(* Logix 5000 AddOnInstructionDefinition export SPEL_LocalSet; software revision 30.01 *)

ADD_ON_INSTRUCTION SPEL_ExecCmd   (* revision 1.2 *)
// Executes a command in the robot controller.  Normally this is called by higher level AOIs.
VAR_INPUT
   Start : BOOL; {required}
   MaxTime : DINT := 3000; {required}
END_VAR
VAR_OUTPUT
   InCycle : BOOL; {access Read Only, visible}
   Done : BOOL; {access Read Only, visible}
   Error : BOOL; {access Read Only, visible}
END_VAR
VAR_IN_OUT
   ExtInputs : AB:ETHERNET_MODULE_INT_128Bytes:I:0; {required}
        .DATA[0].0   // ExtCmdGet
        .DATA[0].1   // ExtRespSet
        .DATA[0].2   // ExtCmdResult
        .DATA[0].3   // ExtError
   ExtOutputs : AB:ETHERNET_MODULE_INT_128Bytes:O:0; {required}
        .DATA[0].0   // ExtCmdSet
        .DATA[0].1   // ExtRespGet
        .DATA[0].2   // ExtCmdReset
END_VAR
VAR_INPUT
   Cmd : INT; {required}
   CmdParam1 : INT; {required}
   CmdParam2 : INT; {required}
   CmdParam3 : INT; {required}
   CmdParam4 : INT; {required}
   CmdParam5 : INT; {required}
   CmdParam6 : INT; {required}
   CmdParam7 : INT; {required}
END_VAR
VAR_OUTPUT
   CmdEcho : INT; {access Read Only, visible}
   Resp1 : INT; {access Read Only, visible}
   Resp2 : INT; {access Read Only, visible}
   Resp3 : INT; {access Read Only, visible}
   Resp4 : INT; {access Read Only, visible}
   Resp5 : INT; {access Read Only, visible}
   Resp6 : INT; {access Read Only, visible}
   Resp7 : INT; {access Read Only, visible}
   ErrCode1 : INT; {access Read Only, visible}
   ErrCode2 : INT; {access Read Only, visible}
END_VAR
VAR
   ExtReset : BOOL; {access None}
   ExtError : BOOL; {access None}
   ExtCmdSet : BOOL; {access None}   // Cmd Ready
   ExtCmdGet : BOOL; {access None}   // Cmd Received
   CmdXferDone : BOOL; {access None}
   ExtRespSet : BOOL; {access None}   // Resp Ready
   RespXferDone : BOOL; {access None}
   ExtCmdResult : BOOL; {access None}   // Normal or Error?
   TmrCmdDataRdy : TIMER := (PRE := 5); {access None}
   OneShotDoneOff : BOOL; {access None}
   OneShotStart : BOOL; {access None}
   StartInit : BOOL; {access None}
   OneShotStartError : BOOL; {access None}
   TmrCycle : TIMER := (PRE := 5000); {access None}
   OneshotTmrPreset : BOOL; {access None}
   TmrCmdSet : TIMER := (PRE := 20); {access None}
   OnShotCmdDataXfer : BOOL; {access None}
   OneShotRespDataXfer : BOOL; {access None}
   OneShotDataRdy : BOOL; {access None}
   OtherCmdInCycle : BOOL; {access None}
   s : BOOL; {access None}
   OneShotUnsetCmdIncycle : BOOL; {access None}
   OneShotSetCmdIncycle : BOOL; {access None}
   OneShotSetOtherCmdInCycleError : BOOL; {access None}
   OneShotSetBit : BOOL; {access None}
   MaxTimeError : BOOL; {access None}
END_VAR

ROUTINE Logic   (* ladder *)
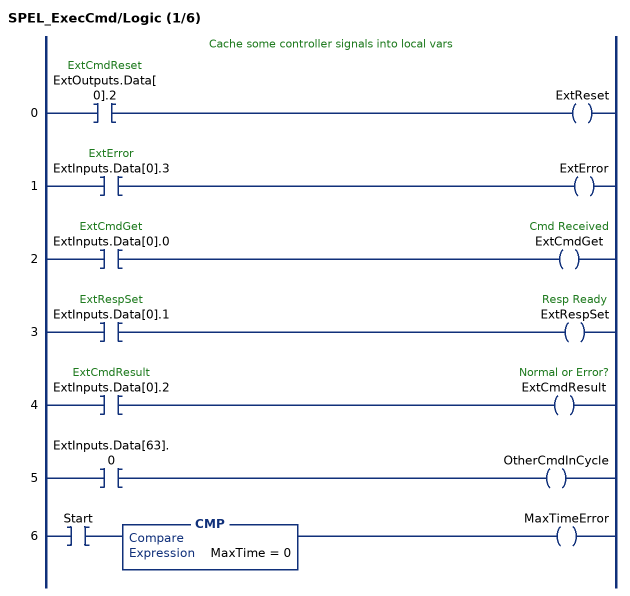
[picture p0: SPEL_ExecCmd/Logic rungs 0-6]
   // Cache some controller signals into local vars
   0: XIC(ExtOutputs.Data[0].2)OTE(ExtReset);
   1: XIC(ExtInputs.Data[0].3)OTE(ExtError);
   2: XIC(ExtInputs.Data[0].0)OTE(ExtCmdGet);
   3: XIC(ExtInputs.Data[0].1)OTE(ExtRespSet);
   4: XIC(ExtInputs.Data[0].2)OTE(ExtCmdResult);
   5: XIC(ExtInputs.Data[63].0)OTE(OtherCmdInCycle);
   6: XIC(Start)CMP(MaxTime = 0)OTE(MaxTimeError);
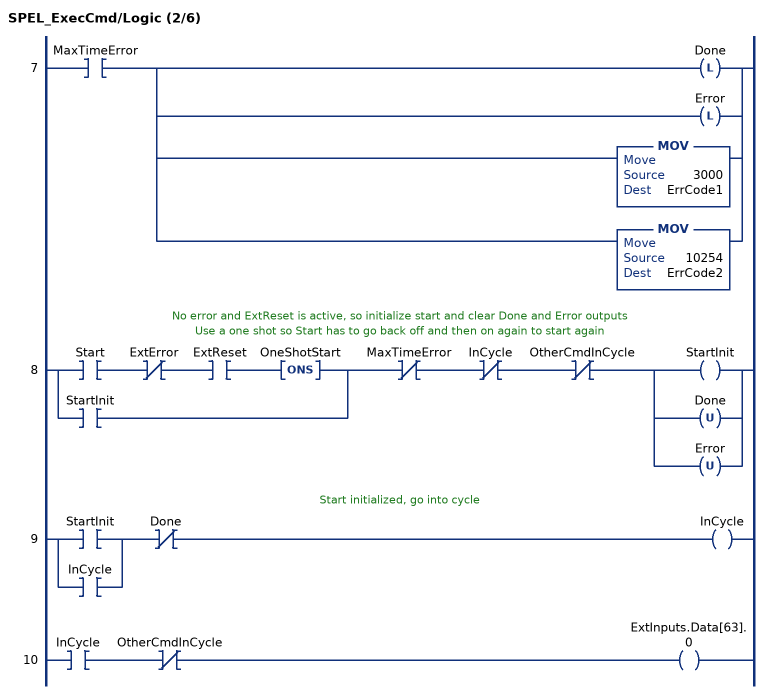
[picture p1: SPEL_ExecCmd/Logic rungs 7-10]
   7: XIC(MaxTimeError)[OTL(Done) ,OTL(Error) ,MOV(3000,ErrCode1) ,MOV(10254,ErrCode2) ];
   // No error and ExtReset is active, so initialize start and clear Done and Error outputs
   // Use a one shot so Start has to go back off and then on again to start again
   8: [XIC(Start) XIO(ExtError) XIC(ExtReset) ONS(OneShotStart) ,XIC(StartInit) ]XIO(MaxTimeError)XIO(InCycle)XIO(OtherCmdInCycle)[OTE(StartInit) ,OTU(Done) ,OTU(Error) ];
   // Start initialized, go into cycle
   9: [XIC(StartInit) ,XIC(InCycle) ]XIO(Done)OTE(InCycle);
   10: XIC(InCycle)XIO(OtherCmdInCycle)OTE(ExtInputs.Data[63].0);
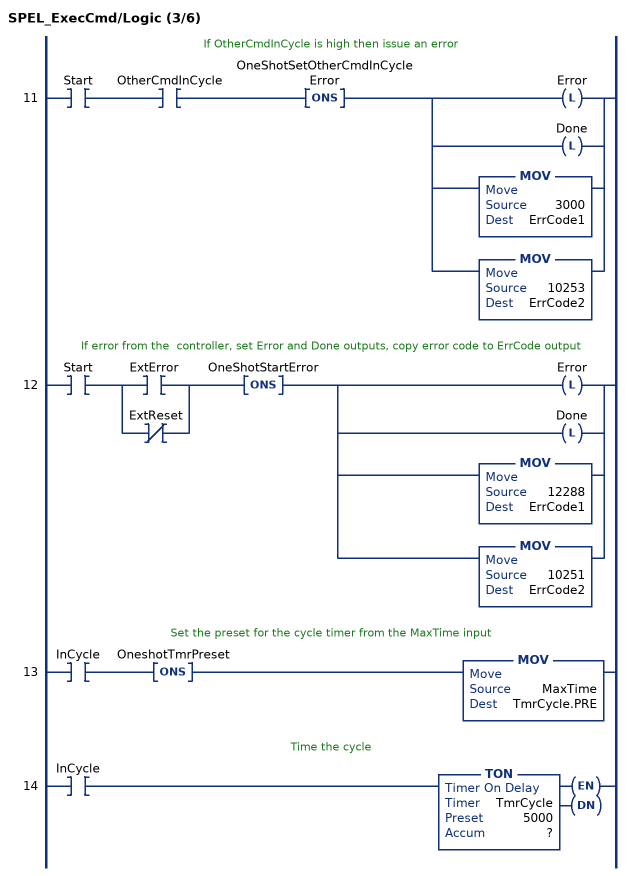
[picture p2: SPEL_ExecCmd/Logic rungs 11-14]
   // If OtherCmdInCycle is high then issue an error
   11: XIC(Start)XIC(OtherCmdInCycle)ONS(OneShotSetOtherCmdInCycleError)[OTL(Error) ,OTL(Done) ,MOV(3000,ErrCode1) ,MOV(10253,ErrCode2) ];
   // If error from the  controller, set Error and Done outputs, copy error code to ErrCode output
   12: XIC(Start)[XIC(ExtError) ,XIO(ExtReset) ]ONS(OneShotStartError)[OTL(Error) ,OTL(Done) ,MOV(12288,ErrCode1) ,MOV(10251,ErrCode2) ];
   // Set the preset for the cycle timer from the MaxTime input
   13: XIC(InCycle)ONS(OneshotTmrPreset)MOV(MaxTime,TmrCycle.PRE);
   // Time the cycle
   14: XIC(InCycle)TON(TmrCycle,?,?);
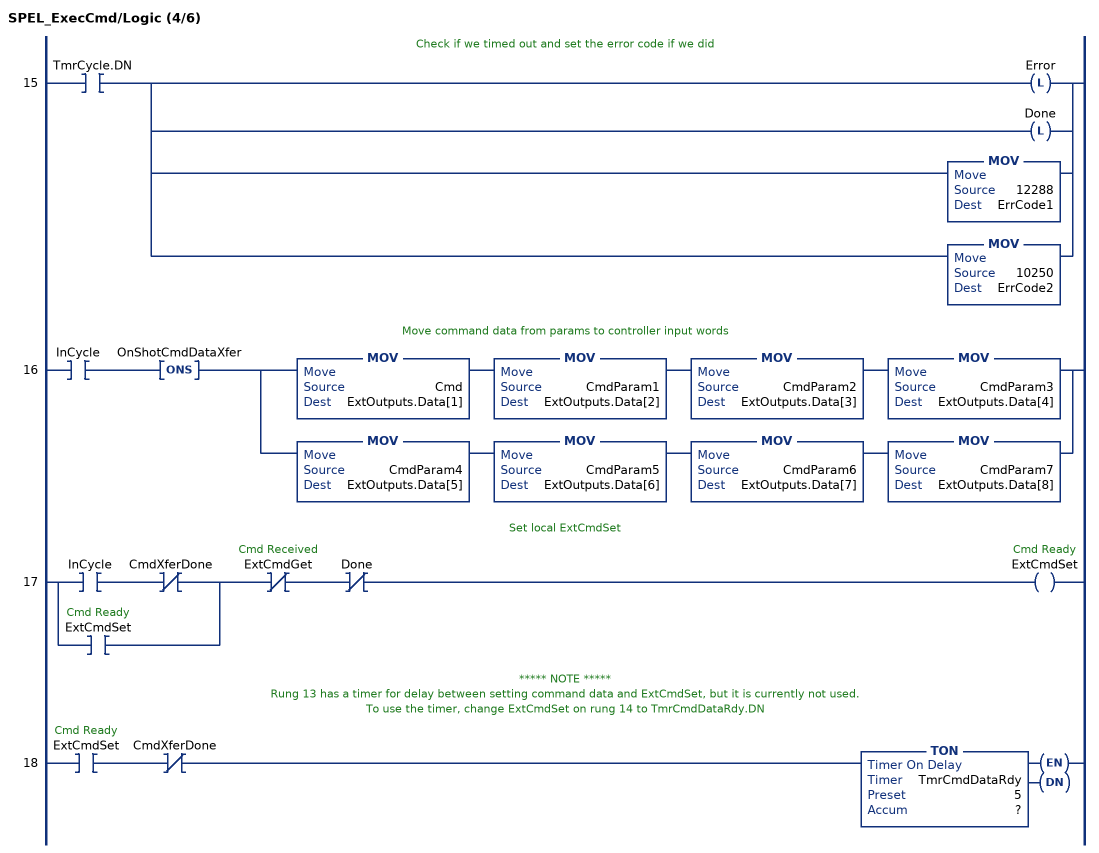
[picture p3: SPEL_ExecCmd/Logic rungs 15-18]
   // Check if we timed out and set the error code if we did
   15: XIC(TmrCycle.DN)[OTL(Error) ,OTL(Done) ,MOV(12288,ErrCode1) ,MOV(10250,ErrCode2) ];
   // Move command data from params to controller input words
   16: XIC(InCycle)ONS(OnShotCmdDataXfer)[MOV(Cmd,ExtOutputs.Data[1]) MOV(CmdParam1,ExtOutputs.Data[2]) MOV(CmdParam2,ExtOutputs.Data[3]) MOV(CmdParam3,ExtOutputs.Data[4]) ,MOV(CmdParam4,ExtOutputs.Data[5]) MOV(CmdParam5,ExtOutputs.Data[6]) MOV(CmdParam6,ExtOutputs.Data[7]) MOV(CmdParam7,ExtOutputs.Data[8]) ];
   // Set local ExtCmdSet
   17: [XIC(InCycle) XIO(CmdXferDone) ,XIC(ExtCmdSet) ]XIO(ExtCmdGet)XIO(Done)OTE(ExtCmdSet);
   // ***** NOTE *****
   // Rung 13 has a timer for delay between setting command data and ExtCmdSet, but it is currently not used.
   // To use the timer, change ExtCmdSet on rung 14 to TmrCmdDataRdy.DN
   18: XIC(ExtCmdSet)XIO(CmdXferDone)TON(TmrCmdDataRdy,?,?);
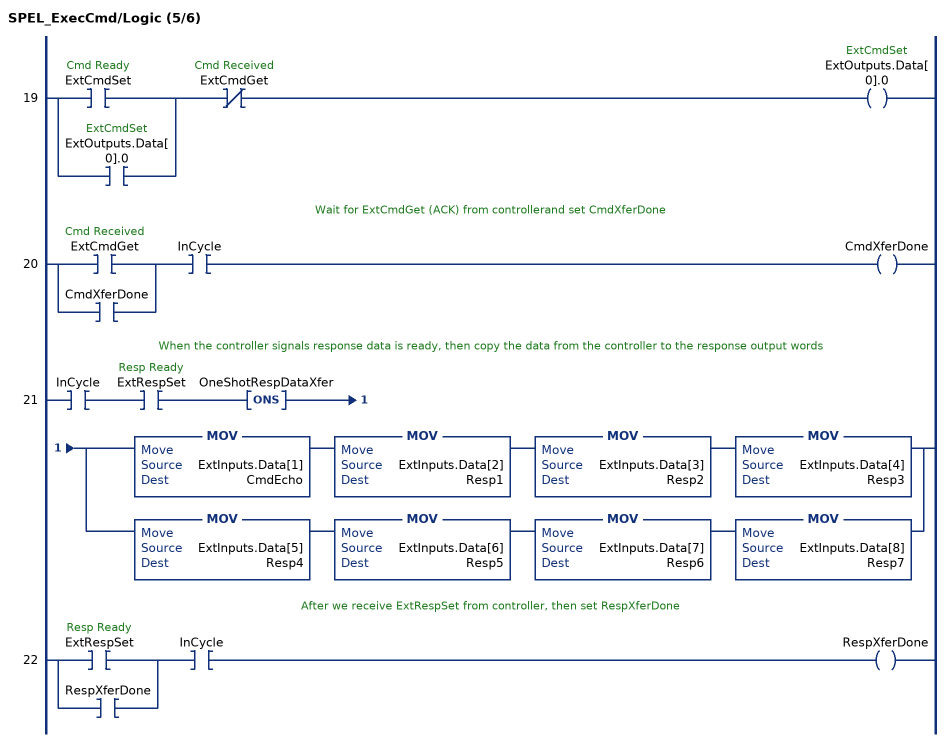
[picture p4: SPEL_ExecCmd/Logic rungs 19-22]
   19: [XIC(ExtCmdSet) ,XIC(ExtOutputs.Data[0].0) ]XIO(ExtCmdGet)OTE(ExtOutputs.Data[0].0);
   // Wait for ExtCmdGet (ACK) from controllerand set CmdXferDone
   20: [XIC(ExtCmdGet) ,XIC(CmdXferDone) ]XIC(InCycle)OTE(CmdXferDone);
   // When the controller signals response data is ready, then copy the data from the controller to the response output words
   21: XIC(InCycle)XIC(ExtRespSet)ONS(OneShotRespDataXfer)[MOV(ExtInputs.Data[1],CmdEcho) MOV(ExtInputs.Data[2],Resp1) MOV(ExtInputs.Data[3],Resp2) MOV(ExtInputs.Data[4],Resp3) ,MOV(ExtInputs.Data[5],Resp4) MOV(ExtInputs.Data[6],Resp5) MOV(ExtInputs.Data[7],Resp6) MOV(ExtInputs.Data[8],Resp7) ];
   // After we receive ExtRespSet from controller, then set RespXferDone
   22: [XIC(ExtRespSet) ,XIC(RespXferDone) ]XIC(InCycle)OTE(RespXferDone);
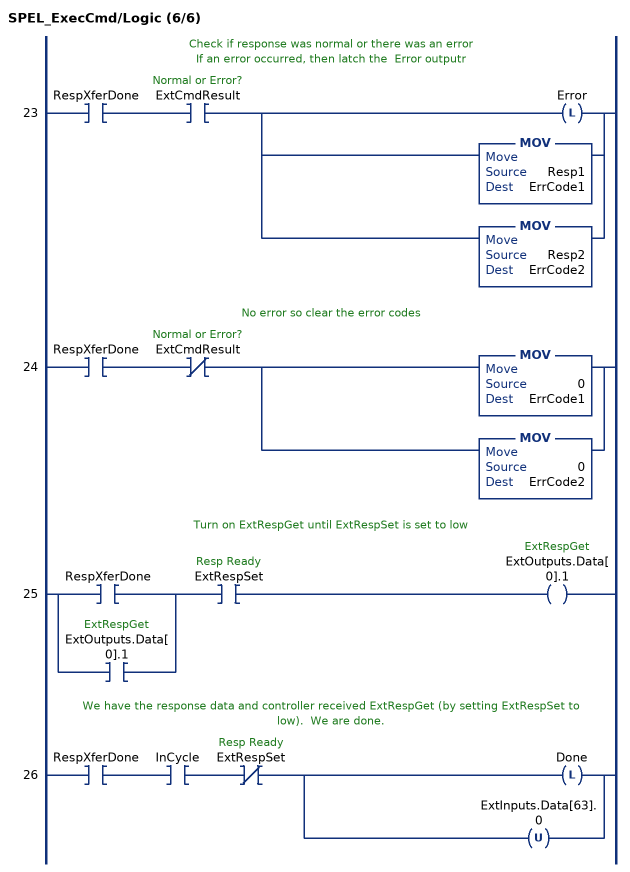
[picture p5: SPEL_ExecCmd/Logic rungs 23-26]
   // Check if response was normal or there was an error
   // If an error occurred, then latch the  Error outputr
   23: XIC(RespXferDone)XIC(ExtCmdResult)[OTL(Error) ,MOV(Resp1,ErrCode1) ,MOV(Resp2,ErrCode2) ];
   // No error so clear the error codes
   24: XIC(RespXferDone)XIO(ExtCmdResult)[MOV(0,ErrCode1) ,MOV(0,ErrCode2) ];
   // Turn on ExtRespGet until ExtRespSet is set to low
   25: [XIC(RespXferDone) ,XIC(ExtOutputs.Data[0].1) ]XIC(ExtRespSet)OTE(ExtOutputs.Data[0].1);
   // We have the response data and controller received ExtRespGet (by setting ExtRespSet to low).  We are done.
   26: XIC(RespXferDone)XIC(InCycle)XIO(ExtRespSet)[OTL(Done) ,OTU(ExtInputs.Data[63].0) ];
END_ROUTINE
END_ADD_ON_INSTRUCTION

ADD_ON_INSTRUCTION SPEL_LocalSet   (* revision 1.2, vendor SEIKO EPSON CORP. *)
// Sets the local coordinate system of the specified coordinate number by each coordinate.
VAR_INPUT
   Start : BOOL; {required}
END_VAR
VAR_OUTPUT
   InCycle : BOOL; {access Read Only, visible}
   Done : BOOL; {access Read Only, visible}
   Error : BOOL; {access Read Only, visible}
END_VAR
VAR_INPUT
   NumAxes : INT; {required}
   LocalNum : INT; {required}
   LocalX : REAL; {required}
   LocalY : REAL; {required}
   LocalZ : REAL; {required}
   LocalU : REAL; {required}
   LocalV : REAL; {required}
   LocalW : REAL; {required}
END_VAR
VAR_IN_OUT
   ExtInputs : AB:ETHERNET_MODULE_INT_128Bytes:I:0; {required}
   ExtOutputs : AB:ETHERNET_MODULE_INT_128Bytes:O:0; {required}
END_VAR
VAR_OUTPUT
   ErrCode1 : INT; {access Read Only, visible}
   ErrCode2 : INT; {access Read Only, visible}
END_VAR
VAR
   Coordinatex1000 : DINT; {access None}
   Coordinate_INTS : INT[2]; {access None}
   ExecLocalSetZ : SPEL_ExecCmd := (MaxTime := 3000); {access None}
   ExecLocalSetY : SPEL_ExecCmd := (MaxTime := 3000); {access None}
   ExecLocalSetX : SPEL_ExecCmd := (MaxTime := 3000); {access None}
   X6 : BOOL; {access None}
   StartInit : BOOL[32]; {access None}
   OneShotStart : BOOL[32]; {access None}
   ExecLocalSetW : SPEL_ExecCmd := (MaxTime := 3000); {access None}
   ExecLocalSetV : SPEL_ExecCmd := (MaxTime := 3000); {access None}
   ExecLocalSetU : SPEL_ExecCmd := (MaxTime := 3000); {access None}
   ExecTimeout : DINT; {access None}
END_VAR

ROUTINE Logic   (* ladder *)
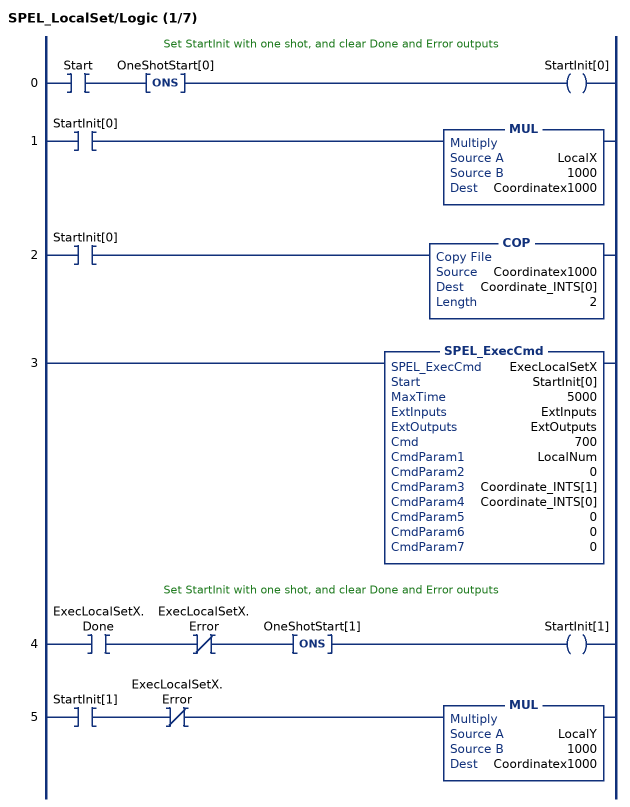
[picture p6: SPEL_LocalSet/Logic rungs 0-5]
   // Set StartInit with one shot, and clear Done and Error outputs
   0: XIC(Start)ONS(OneShotStart[0])OTE(StartInit[0]);
   1: XIC(StartInit[0])MUL(LocalX,1000,Coordinatex1000);
   2: XIC(StartInit[0])COP(Coordinatex1000,Coordinate_INTS[0],2);
   3: SPEL_ExecCmd(ExecLocalSetX,StartInit[0],5000,ExtInputs,ExtOutputs,700,LocalNum,0,Coordinate_INTS[1],Coordinate_INTS[0],0,0,0);
   // Set StartInit with one shot, and clear Done and Error outputs
   4: XIC(ExecLocalSetX.Done)XIO(ExecLocalSetX.Error)ONS(OneShotStart[1])OTE(StartInit[1]);
   5: XIC(StartInit[1])XIO(ExecLocalSetX.Error)MUL(LocalY,1000,Coordinatex1000);
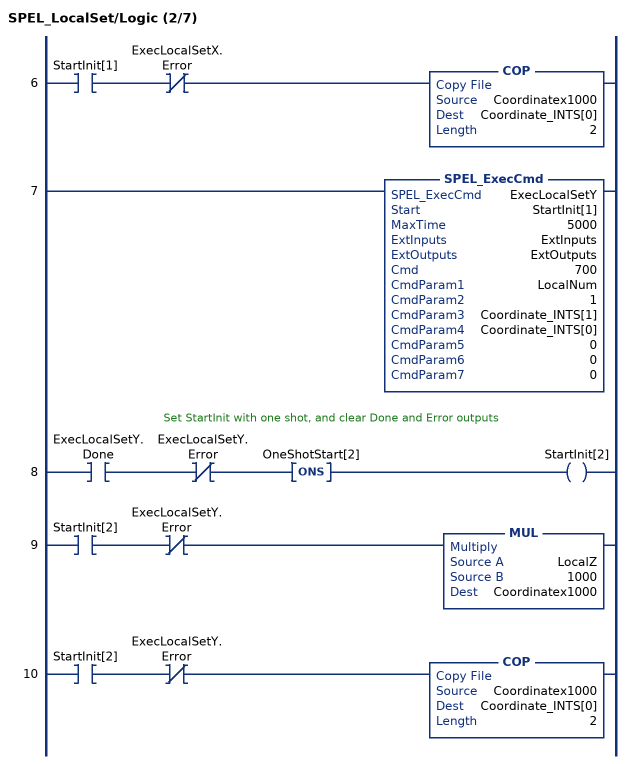
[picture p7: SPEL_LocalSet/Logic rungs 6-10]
   6: XIC(StartInit[1])XIO(ExecLocalSetX.Error)COP(Coordinatex1000,Coordinate_INTS[0],2);
   7: SPEL_ExecCmd(ExecLocalSetY,StartInit[1],5000,ExtInputs,ExtOutputs,700,LocalNum,1,Coordinate_INTS[1],Coordinate_INTS[0],0,0,0);
   // Set StartInit with one shot, and clear Done and Error outputs
   8: XIC(ExecLocalSetY.Done)XIO(ExecLocalSetY.Error)ONS(OneShotStart[2])OTE(StartInit[2]);
   9: XIC(StartInit[2])XIO(ExecLocalSetY.Error)MUL(LocalZ,1000,Coordinatex1000);
   10: XIC(StartInit[2])XIO(ExecLocalSetY.Error)COP(Coordinatex1000,Coordinate_INTS[0],2);
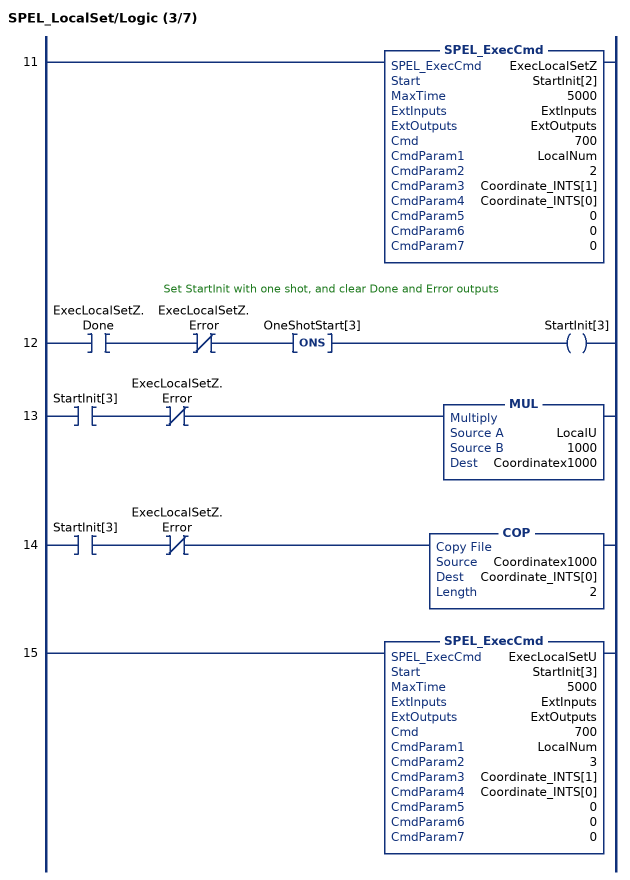
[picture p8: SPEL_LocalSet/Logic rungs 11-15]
   11: SPEL_ExecCmd(ExecLocalSetZ,StartInit[2],5000,ExtInputs,ExtOutputs,700,LocalNum,2,Coordinate_INTS[1],Coordinate_INTS[0],0,0,0);
   // Set StartInit with one shot, and clear Done and Error outputs
   12: XIC(ExecLocalSetZ.Done)XIO(ExecLocalSetZ.Error)ONS(OneShotStart[3])OTE(StartInit[3]);
   13: XIC(StartInit[3])XIO(ExecLocalSetZ.Error)MUL(LocalU,1000,Coordinatex1000);
   14: XIC(StartInit[3])XIO(ExecLocalSetZ.Error)COP(Coordinatex1000,Coordinate_INTS[0],2);
   15: SPEL_ExecCmd(ExecLocalSetU,StartInit[3],5000,ExtInputs,ExtOutputs,700,LocalNum,3,Coordinate_INTS[1],Coordinate_INTS[0],0,0,0);
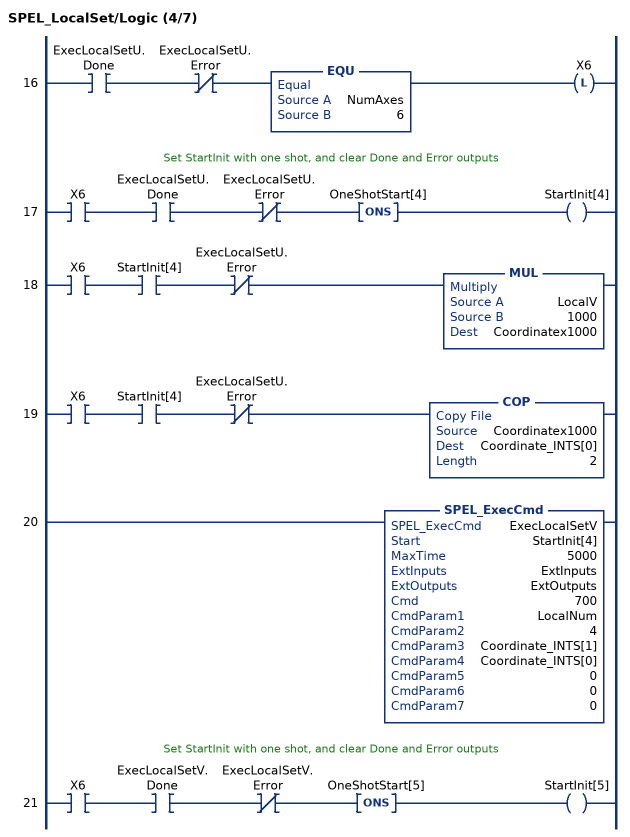
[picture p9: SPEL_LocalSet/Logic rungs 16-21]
   16: XIC(ExecLocalSetU.Done)XIO(ExecLocalSetU.Error)EQU(NumAxes,6)OTL(X6);
   // Set StartInit with one shot, and clear Done and Error outputs
   17: XIC(X6)XIC(ExecLocalSetU.Done)XIO(ExecLocalSetU.Error)ONS(OneShotStart[4])OTE(StartInit[4]);
   18: XIC(X6)XIC(StartInit[4])XIO(ExecLocalSetU.Error)MUL(LocalV,1000,Coordinatex1000);
   19: XIC(X6)XIC(StartInit[4])XIO(ExecLocalSetU.Error)COP(Coordinatex1000,Coordinate_INTS[0],2);
   20: SPEL_ExecCmd(ExecLocalSetV,StartInit[4],5000,ExtInputs,ExtOutputs,700,LocalNum,4,Coordinate_INTS[1],Coordinate_INTS[0],0,0,0);
   // Set StartInit with one shot, and clear Done and Error outputs
   21: XIC(X6)XIC(ExecLocalSetV.Done)XIO(ExecLocalSetV.Error)ONS(OneShotStart[5])OTE(StartInit[5]);
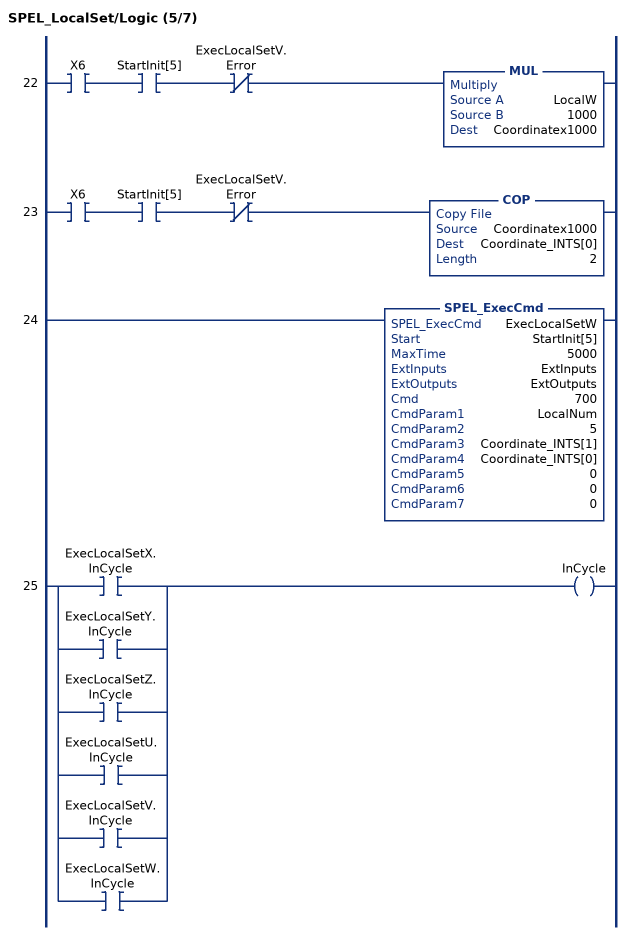
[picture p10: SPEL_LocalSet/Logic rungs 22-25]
   22: XIC(X6)XIC(StartInit[5])XIO(ExecLocalSetV.Error)MUL(LocalW,1000,Coordinatex1000);
   23: XIC(X6)XIC(StartInit[5])XIO(ExecLocalSetV.Error)COP(Coordinatex1000,Coordinate_INTS[0],2);
   24: SPEL_ExecCmd(ExecLocalSetW,StartInit[5],5000,ExtInputs,ExtOutputs,700,LocalNum,5,Coordinate_INTS[1],Coordinate_INTS[0],0,0,0);
   25: [XIC(ExecLocalSetX.InCycle) ,XIC(ExecLocalSetY.InCycle) ,XIC(ExecLocalSetZ.InCycle) ,XIC(ExecLocalSetU.InCycle) ,XIC(ExecLocalSetV.InCycle) ,XIC(ExecLocalSetW.InCycle) ]OTE(InCycle);
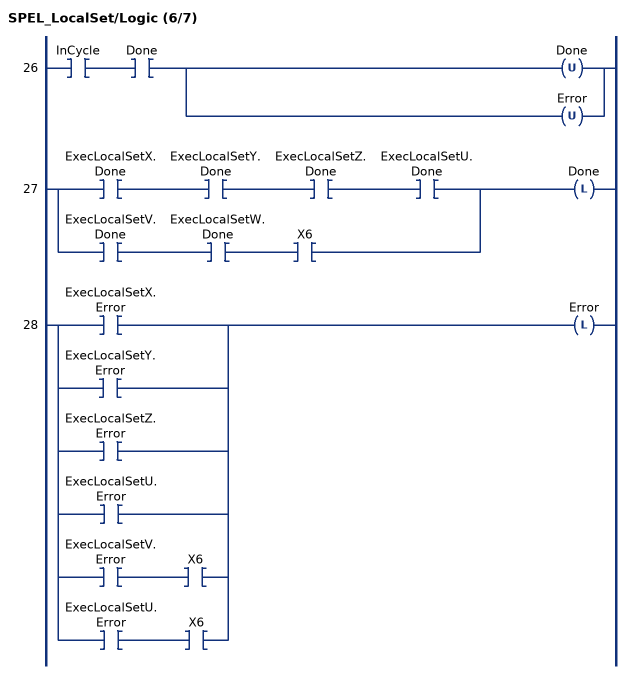
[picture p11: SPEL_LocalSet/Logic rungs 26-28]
   26: XIC(InCycle)XIC(Done)[OTU(Done) ,OTU(Error) ];
   27: [XIC(ExecLocalSetX.Done) XIC(ExecLocalSetY.Done) XIC(ExecLocalSetZ.Done) XIC(ExecLocalSetU.Done) ,XIC(ExecLocalSetV.Done) XIC(ExecLocalSetW.Done) XIC(X6) ]OTL(Done);
   28: [XIC(ExecLocalSetX.Error) ,XIC(ExecLocalSetY.Error) ,XIC(ExecLocalSetZ.Error) ,XIC(ExecLocalSetU.Error) ,XIC(ExecLocalSetV.Error) XIC(X6) ,XIC(ExecLocalSetU.Error) XIC(X6) ]OTL(Error);
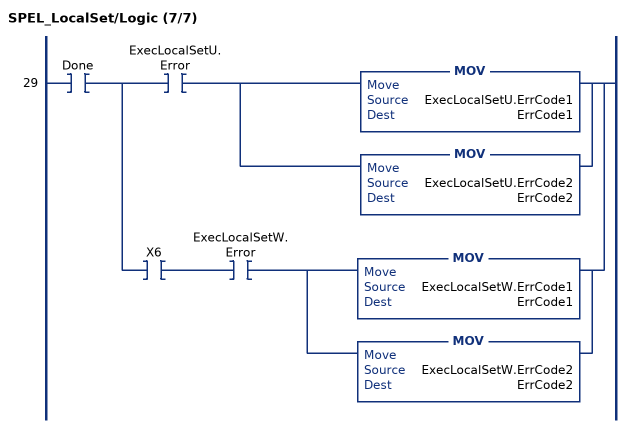
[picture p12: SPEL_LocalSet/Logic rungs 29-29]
   29: XIC(Done)[XIC(ExecLocalSetU.Error) [MOV(ExecLocalSetU.ErrCode1,ErrCode1) ,MOV(ExecLocalSetU.ErrCode2,ErrCode2) ] ,XIC(X6) XIC(ExecLocalSetW.Error) [MOV(ExecLocalSetW.ErrCode1,ErrCode1) ,MOV(ExecLocalSetW.ErrCode2,ErrCode2) ] ];
END_ROUTINE
END_ADD_ON_INSTRUCTION
